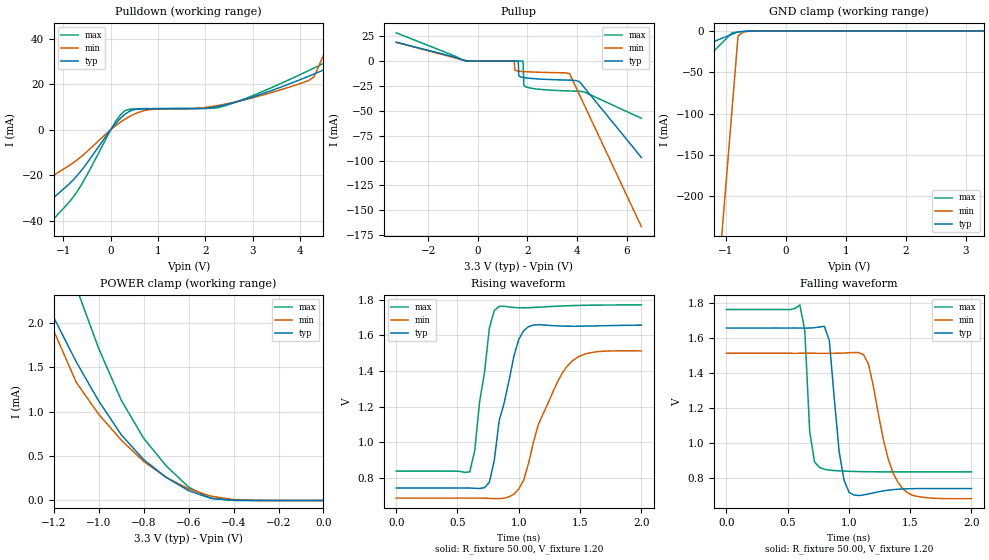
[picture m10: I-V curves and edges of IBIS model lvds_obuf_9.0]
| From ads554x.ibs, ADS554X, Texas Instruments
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|   Model lvds_obuf_9.0
[Model]   lvds_obuf_9.0
Model_type   3-state
Polarity   Non-Inverting
Enable   Active-High
Vmeas =   1.2000V
Cref =   5.0000pF
Rref = 50.0000
Vref =   1.2000V
C_comp   2.13pF   1.93pF   2.33pF
[Temperature Range]   27.00   125   -40.00
[Voltage Range]   3.30V   3.00V   3.60V
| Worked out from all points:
|   slope of the pulldown table from 0 to 0.495 V, typ, clamps not added: 55.8 ohm
|   slope of the pullup table from 0 to 0.495 V, typ, clamps not added: 76.7 kohm
|   GND clamp passes 1 mA (typ) near -0.79 V on its own axis
|   POWER clamp passes 1 mA (typ) near -0.97 V on its own axis
|   rising waveform, R_fixture 50.00, V_fixture 1.20: 20-80 % time 152ps typ, 255ps min, 100ps max; typ from 0.743 V to 1.66 V
|   falling waveform, R_fixture 50.00, V_fixture 1.20: 20-80 % time 73.4ps typ, 158ps min, 45.9ps max; typ from 1.66 V to 0.742 V
[Pulldown]
| voltage   I(typ)   I(min)   I(max)
-3.3V     -67.96mA   -47.02mA   -85.65mA
-2.1V     -46.12mA   -31.54mA   -59.01mA
-1.5V     -35.2mA    -23.8mA    -45.69mA
-700mV    -19.97mA   -13.12mA   -26.89mA
300mV     6.73mA     4.59mA     8.31mA
2.3V      10.31mA    10.76mA    9.82mA
4.2V      23.6mA     21.73mA    26.08mA
4.7V      28.11mA    42.12mA    31.11mA
4.9V      34.36mA    51.58mA    33.16mA
5.1V      53.31mA    61.04mA    35.4mA
5.3V      72.26mA    70.5mA     44.49mA
6.6V      195.4mA    132mA      184.8mA
[Pullup]
| voltage   I(typ)   I(min)   I(max)
-3.3V     18.99mA    18.89mA    28.44mA
-500mV    380uA      570uA      360uA
1.46V     51.1uA     6.307uA    77.46uA
1.62V     11.84uA    -10.01mA   68.15uA
1.66V     -14.79mA   -10.12mA   65.81uA
1.81V     -16.42mA   -10.46mA   50.28uA
1.83V     -16.49mA   -10.5mA    -3.55mA
1.85V     -16.57mA   -10.53mA   -22.39mA
1.9V      -16.74mA   -10.62mA   -25.43mA
3.7V      -19.13mA   -12.64mA   -30.02mA
4.1V      -20.61mA   -33.84mA   -30.33mA
6.6V      -96.86mA   -166.3mA   -57.45mA
[GND_clamp]
| voltage   I(typ)   I(min)   I(max)
-3.3V     -73.53mA   -2.228A    -176.7mA
-1.1V     -9.73mA    -272.6mA   -16.77mA
-1V       -6.83mA    -183.7mA   -9.5mA
-900mV    -3.93mA    -94.8mA    -2.23mA
-800mV    -1.03mA    -5.92mA    -1.19mA
-700mV    -450uA     -730uA     -490uA
3.3V      44.64pA    1.08uA     37.43pA
[POWER_clamp]
| voltage   I(typ)   I(min)   I(max)
-3.3V     247.8mA    491.9mA    558.7mA
-1.3V     2.62mA     3.21mA     3.99mA
-1.2V     2.06mA     1.91mA     3.16mA
-1.1V     1.56mA     1.33mA     2.4mA
-1V       1.12mA     970uA      1.71mA
-900mV    740uA      680uA      1.13mA
-800mV    460uA      440uA      700uA
-700mV    260uA      260uA      390uA
-600mV    110uA      130uA      150uA
-500mV    23.34uA    48.47uA    24.97uA
-400mV    2uA        9.55uA     1.31uA
0V        44.64pA    500pA      43.31pA
[Ramp]
| variable   typ   min   max
dV/dt_r   1.84/71.03p   1.61/0.12n   2.05/47.00p
dV/dt_f   1.84/94.06p   1.65/0.14n   2.00/0.12n
R_load = 1.00k
[Rising Waveform]
R_fixture = 50.00
V_fixture = 1.20
V_fixture_min = 1.10
V_fixture_max = 1.30
| time   V(typ)   V(min)   V(max)
0s        743.1mV    686.5mV    837.5mV
600ps     743.1mV    686.6mV    833.6mV
640ps     741.3mV    686.5mV    949.9mV
760ps     775.2mV    685mV      1.64V
840ps     1.121V     683.1mV    1.761V
1ns       1.577V     737.7mV    1.754V
1.08ns    1.648V     882.4mV    1.754V
1.16ns    1.659V     1.1V       1.757V
1.4ns     1.651V     1.431V     1.765V
2ns       1.657V     1.512V     1.77V
[Falling Waveform]
R_fixture = 50.00
V_fixture = 1.20
V_fixture_min = 1.10
V_fixture_max = 1.30
| time   V(typ)   V(min)   V(max)
0s        1.657V     1.513V     1.763V
600ps     1.657V     1.513V     1.789V
640ps     1.657V     1.513V     1.642V
680ps     1.657V     1.513V     1.068V
760ps     1.663V     1.513V     863.1mV
840ps     1.587V     1.513V     847.6mV
1ns       722.5mV    1.516V     840.9mV
1.16ns    711.6mV    1.451V     838.4mV
1.44ns    740.1mV    741.1mV    837.5mV
2ns       742.4mV    684.8mV    837.4mV
